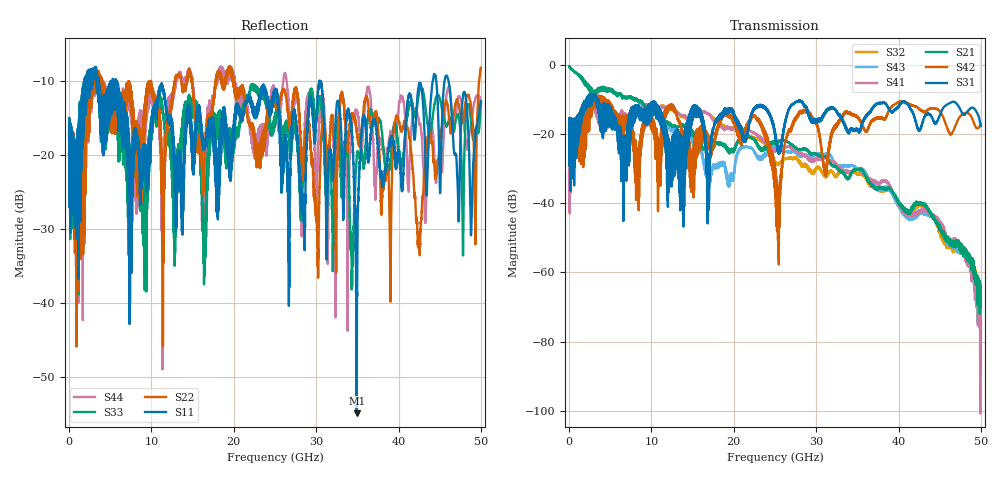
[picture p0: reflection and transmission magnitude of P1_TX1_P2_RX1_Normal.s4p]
!Keysight Technologies,N5225A,MY51441389,A.10.49.11
!Date: Monday, July 08, 2019 10:52:27
!Correction: S11(Full 4 Port(1,2,3,4))
!S12(Full 4 Port(1,2,3,4))
!S13(Full 4 Port(1,2,3,4))
!S14(Full 4 Port(1,2,3,4))
!S21(Full 4 Port(1,2,3,4))
!S22(Full 4 Port(1,2,3,4))
!S23(Full 4 Port(1,2,3,4))
!S24(Full 4 Port(1,2,3,4))
!S31(Full 4 Port(1,2,3,4))
!S32(Full 4 Port(1,2,3,4))
!S33(Full 4 Port(1,2,3,4))
!S34(Full 4 Port(1,2,3,4))
!S41(Full 4 Port(1,2,3,4))
!S42(Full 4 Port(1,2,3,4))
!S43(Full 4 Port(1,2,3,4))
!S44(Full 4 Port(1,2,3,4))
!S4P File: Measurements: <S11,S12,S13,S14>,
!<S21,S22,S23,S24>,
!<S31,S32,S33,S34>,
!<S41,S42,S43,S44>:
# Hz S  dB  R 50
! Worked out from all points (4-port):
!   5000 points, 10 MHz to 50 GHz, reference 50 ohm
!   strongest paths, dB at 10 MHz, 12.51 GHz, 25.01 GHz, 37.51 GHz, 50 GHz:
!     S31: -19.1, -22.5, -19.9, -11.2, -17.7
!     S42: -19.1, -12.4, -36.7, -15.3, -17.2
!     S21: -0.4, -17.9, -22.2, -35.6, -67.3
!     S41: -32.9, -12.7, -24.4, -34.2, -72.9
!     S43: -0.4, -19.4, -23.5, -36.1, -89.3
!     S32: -33.1, -12.9, -27.9, -36.2, -78.8
!   lowest |S11| = -54.9 dB at 34.93 GHz (marker M1), VSWR 1.00, Z = 49.9 - j0.168 ohm
!   |S11| at or under -10 dB: start of sweep to 1.93 GHz; 5.702 GHz to 44.15 GHz (38.45 GHz wide, 154 % of centre); 46.07 GHz to end of sweep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
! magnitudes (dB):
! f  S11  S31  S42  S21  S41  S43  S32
! 10 MHz  -17.4  -19.1  -19.1  -0.4  -32.9  -0.4  -33.1
! 2.31 GHz  -11.3  -10.5  -14.3  -6.4  -10.6  -6.4  -10.5
! 16.44 GHz  -18.7  -17.9  -18.6  -24.3  -13.7  -28.9  -13.7
! 22.5 GHz  -14.5  -12.8  -14.6  -21.8  -19.7  -25.1  -21.3
! 25.4 GHz  -14.1  -25.5  -38.7  -22.0  -23.9  -23.8  -28.7
! 34.93 GHz  -54.9  -18.8  -14.9  -30.2  -30.3  -29.9  -31.6
! 50 GHz  -12.8  -17.7  -17.2  -67.3  -72.9  -89.3  -78.8
